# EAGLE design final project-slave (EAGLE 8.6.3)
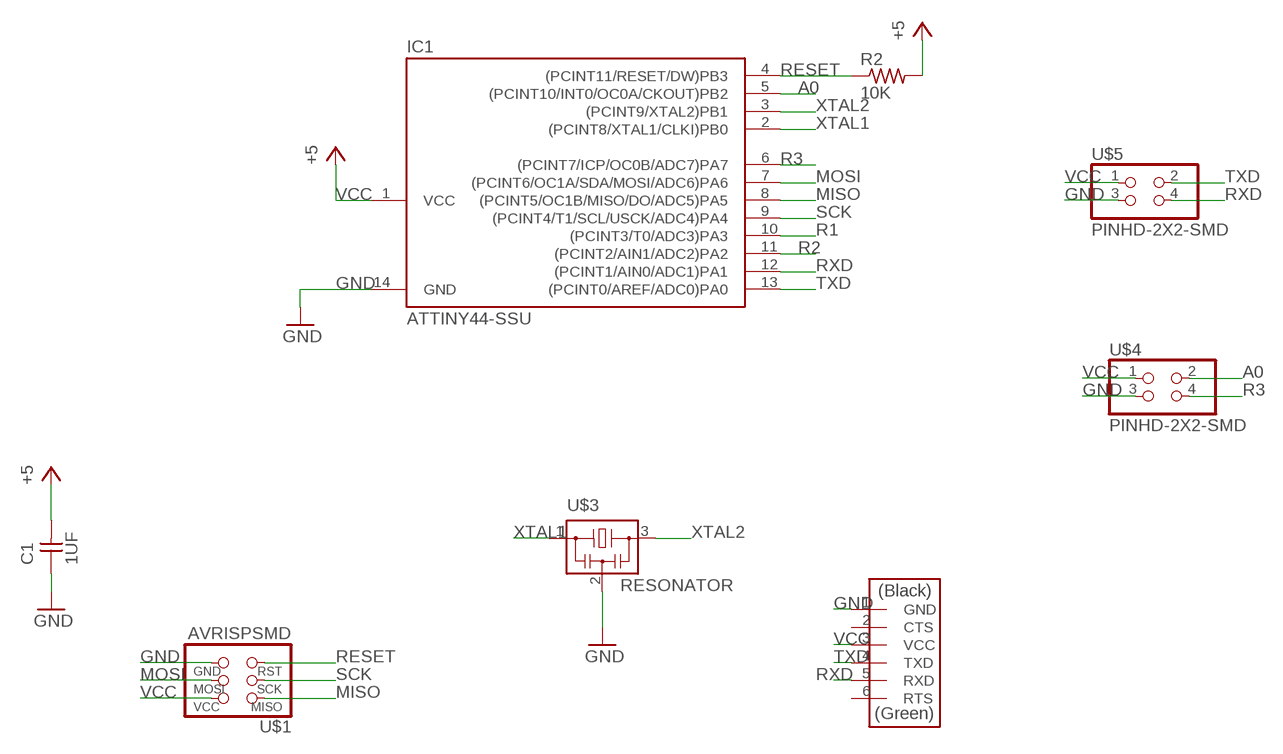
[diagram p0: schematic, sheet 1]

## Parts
C1  1UF  CAP-UNPOLARIZEDFAB  [C1206FAB]
IC1  ATTINY44-SSU  [SOIC14]
R2  10K  RES-US1206FAB  [R1206FAB]
U$1  AVRISPSMD  [2X03SMD]
U$2  FTDI-SMD-HEADER  [1X06SMD]
U$3  RESONATOR  [EFOBM]
U$4  PINHD-2X2-SMD  [2X02SMD]
U$5  PINHD-2X2-SMD  [2X02SMD]

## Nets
A0: IC1.5((PCINT10/INT0/OC0A/CKOUT)PB2) U$4.2
GND: C1.1 IC1.14(GND) U$1.6(GND) U$2.1(GND) U$3.2 U$4.3 U$5.3
MISO: IC1.8((PCINT5/OC1B/MISO/DO/ADC5)PA5) U$1.1(MISO)
MOSI: IC1.7((PCINT6/OC1A/SDA/MOSI/ADC6)PA6) U$1.4(MOSI)
R1: IC1.10((PCINT3/T0/ADC3)PA3)
R2: IC1.11((PCINT2/AIN1/ADC2)PA2)
R3: IC1.6((PCINT7/ICP/OC0B/ADC7)PA7) U$4.4
RESET: IC1.4((PCINT11/RESET/DW)PB3) R2.1 U$1.5(RST)
RXD: IC1.12((PCINT1/AIN0/ADC1)PA1) U$2.5(RXD) U$5.4
SCK: IC1.9((PCINT4/T1/SCL/USCK/ADC4)PA4) U$1.3(SCK)
TXD: IC1.13((PCINT0/AREF/ADC0)PA0) U$2.4(TXD) U$5.2
VCC: C1.2 IC1.1(VCC) R2.2 U$1.2(VCC) U$2.3(VCC) U$4.1 U$5.1 ; supply symbol labelled +5
XTAL1: IC1.2((PCINT8/XTAL1/CLKI)PB0) U$3.1
XTAL2: IC1.3((PCINT9/XTAL2)PB1) U$3.3
Unconnected: U$2.2(CTS) U$2.6(RTS)

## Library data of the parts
C1 = fab:CAP-UNPOLARIZED
IC1 = fab:ATTINY44
R2 = fab:RES-US: Resistor (US Symbol)
U$1 = fab:AVRISP
U$2 = fab:FTDI-SMD-HEADER
U$3 = fab:RESONATOR
U$4 U$5 = fab:PINHD-2X2-SMD

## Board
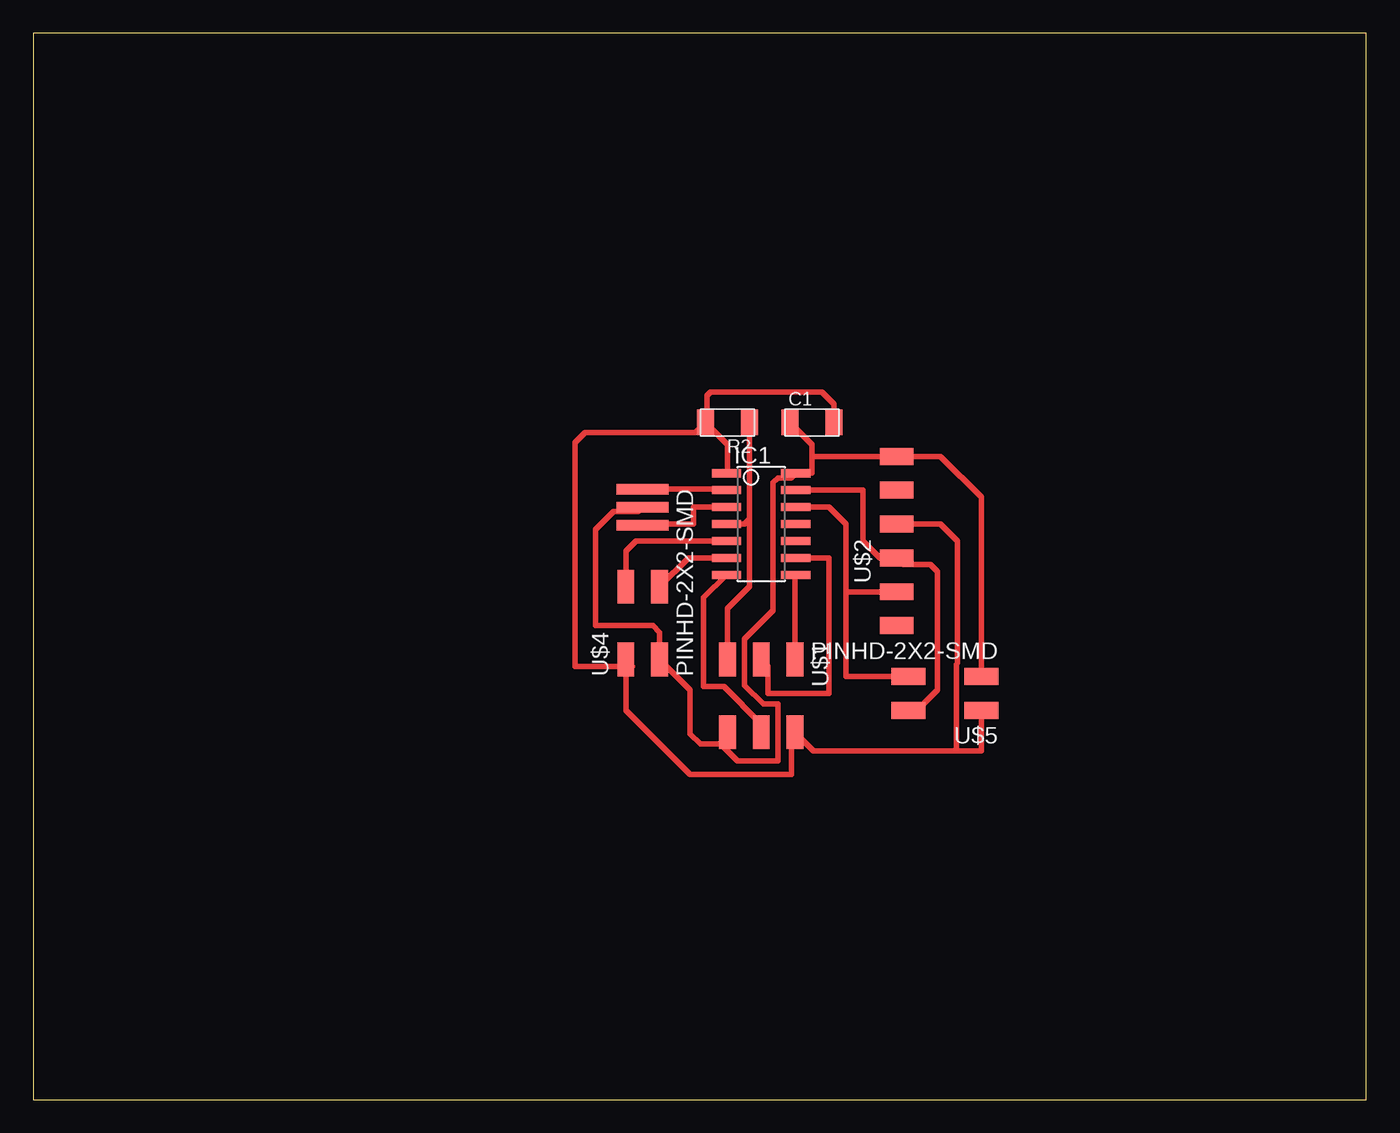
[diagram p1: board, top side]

Size 100 x 80 mm. Coordinates in mm from the lower left corner, seen from the top.
Outline: 0,0 100,0 100,80 0,80 0,0
Copper layers (1*16): Top 0.035mm / dielectric 1.5mm / Bottom 0.035mm
Design rules "rules": minimum track width 16mil, minimum drill 0.8mm, track to track 16mil, track to pad 16mil, pad to pad 16mil, via to via 16mil, smd to smd 16mil, copper to edge 40mil, drill to drill 6mil, minimum pad ring 10mil, minimum via ring 8mil, stop-mask expansion 4mil, vias tented up to drill 0mil, thermal gap 10mil

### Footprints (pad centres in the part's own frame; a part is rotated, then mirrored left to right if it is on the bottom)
C1206FAB = smd 1.27 x 1.905: 1 -1.651,0; 2 1.651,0
SOIC14 = smd 0.61 x 2.21: 1 -3.81,-2.603; 2 -2.54,-2.603; 3 -1.27,-2.603; 4 0,-2.603; 5 1.27,-2.603; 6 2.54,-2.603; 7 3.81,-2.603; 8 3.81,2.603; 9 2.54,2.603; 10 1.27,2.603; 11 0,2.603; 12 -1.27,2.603; 13 -2.54,2.603; 14 -3.81,2.603
R1206FAB = smd 1.27 x 1.905: 1 -1.651,0; 2 1.651,0
2X03SMD = smd 2.54 x 1.27: 1 -2.54,2.54; 2 2.92,2.54; 3 -2.54,0; 4 2.92,0; 5 -2.54,-2.54; 6 2.92,-2.54
1X06SMD = smd 2.54 x 1.27: 1 0,6.35; 2 0,3.81; 3 0,1.27; 4 0,-1.27; 5 0,-3.81; 6 0,-6.35
EFOBM = smd 0.8 x 3.9: 1 -1.35,0; 2 0,0; 3 1.35,0
2X02SMD = smd 2.54 x 1.27: 1 -2.54,1.27; 2 2.92,1.27; 3 -2.54,-1.27; 4 2.92,-1.27

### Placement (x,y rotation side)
C1  58.42,50.8 0 top
IC1  54.61,43.18 270 top
R2  52.07,50.8 180 top
U$1  54.61,30.48 270 top
U$2  64.77,41.91 0 top
U$3  45.72,44.45 270 top
U$4  45.72,35.56 90 top
U$5  68.58,30.48 180 top

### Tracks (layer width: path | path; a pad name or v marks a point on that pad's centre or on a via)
A0
  Top 0.406: IC1.5 45.21,41.91 44.45,41.15 U$4.2
GND
  Top 0.406: 58.42,48.26 U$2.1 68.07,48.26 71.12,45.21 U$5.3 | 58.42,48.26 58.42,46.99 IC1.14 56.86,46.63 55.86,46.63 55.5,46.28 55.5,36.68 53.37,34.54 53.37,31.08 54.78,29.67 55.88,29.67 55.88,25.4 52.83,25.4 51.82,26.42 52.07,26.67 | U$3.2 45.38,44.11 43.52,44.11 42.16,42.76 42.16,35.56 46.48,35.56 46.99,35.05 U$4.3 49.28,30.73 49.28,27.43 50.04,26.67 52.07,26.67 | 52.07,26.67 U$1.6 | C1.1 58.42,49.15 58.42,48.26
MISO
  Top 0.406: IC1.8 57.15,39.31 U$1.1
MOSI
  Top 0.406: IC1.7 50.29,37.66 50.29,30.99 51.82,30.99 54.61,28.19 U$1.4
R3
  Top 0.406: IC1.6 49.15,40.64 U$4.4
RESET
  Top 0.406: R2.1 53.72,43.56 | IC1.4 53.34,43.18 53.72,43.56 | 53.72,43.56 53.72,38.48 52.07,36.83 U$1.5
RXD
  Top 0.406: IC1.12 59.69,44.45 60.96,43.18 60.96,38.1 | 60.96,38.1 U$2.5 | 60.96,38.1 60.96,31.75 U$5.4
SCK
  Top 0.406: IC1.9 59.69,40.64 59.69,30.48 55.12,30.48 55.12,32.51 U$1.3
TXD
  Top 0.406: IC1.13 62.23,45.72 62.23,41.91 63.5,40.64 U$2.4 65.28,40.13 67.31,40.13 67.82,39.62 67.82,30.73 66.29,29.21 U$5.2
VCC
  Top 0.406: 69.09,26.16 58.55,26.16 U$1.2 56.9,27.31 56.9,24.38 49.28,24.38 44.45,29.21 44.45,32.51 | 69.09,26.16 71.12,26.16 U$5.1 | U$2.3 68.07,43.18 69.34,41.91 69.34,32.74 69.24,32.64 69.24,26.31 69.09,26.16 | U$4.1 44.45,32.51 | 44.45,32.51 40.64,32.51 40.64,49.28 41.4,50.04 49.66,50.04 R2.2 50.55,50.67 | 44.96,32.51 44.45,32.51 | IC1.1 52.07,47.05 52.07,49.15 50.61,50.61 50.55,50.67 | C1.2 60.07,52.2 59.18,53.09 50.8,53.09 50.55,52.83 50.55,50.67
XTAL1
  Top 0.406: IC1.2 51.93,45.8 U$3.1
XTAL2
  Top 0.406: IC1.3 49.53,44.45 49.53,43.18 45.8,43.18 U$3.3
